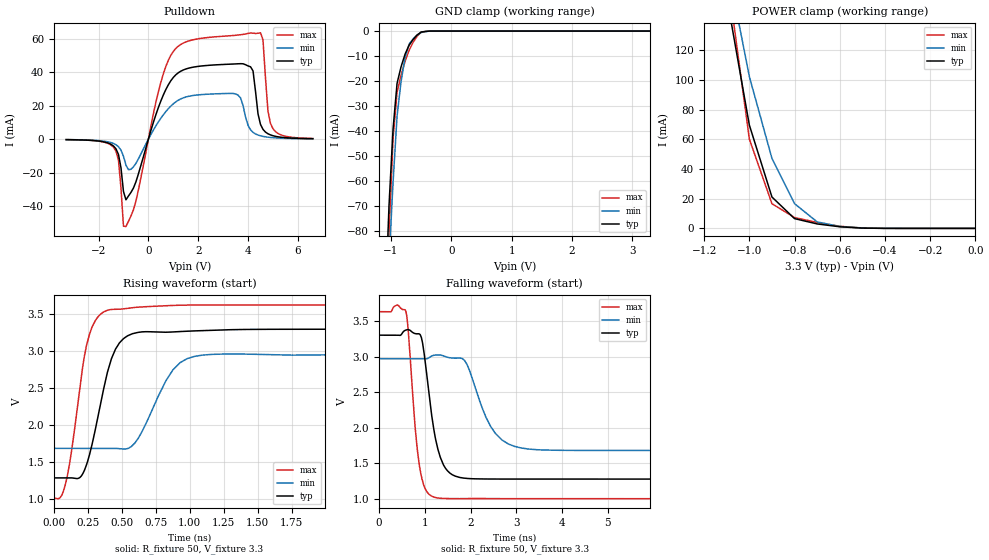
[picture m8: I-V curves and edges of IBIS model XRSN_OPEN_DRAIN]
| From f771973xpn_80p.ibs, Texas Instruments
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|   Model Cell XRSN_OPEN_DRAIN
|XRSN_OPEN_DRAIN
[Model]   XRSN_OPEN_DRAIN
Model_type   I/O_open_drain
Polarity   Non-Inverting
Enable   Active-High
Vinl =  0.8
Vinh =  2
Cref =  15.0000pF
Rref =  100.0000M
Vref =  0V
Vmeas =  1.65
C_comp   4.25494p   0.807076p   4.29559p
[Model Spec]
Vinl   0.8   0.8   0.8
Vinh   2   2   2
[Temperature Range]   25   155   -40
[Voltage Range]   3.3   2.97   3.63
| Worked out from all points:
|   slope of the pulldown table from 0 to 0.495 V, typ, clamps not added: 22 ohm
|   GND clamp passes 1 mA (typ) near -0.53 V on its own axis
|   POWER clamp passes 1 mA (typ) near -0.59 V on its own axis
|   rising waveform, R_fixture 50, V_fixture 3.3: 20-80 % time 149ps typ, 207ps min, 123ps max; typ from 1.28 V to 3.3 V
|   falling waveform, R_fixture 50, V_fixture 3.3: 20-80 % time 278ps typ, 497ps min, 202ps max; typ from 3.3 V to 1.28 V
| Nom Voltages:
|   BIASFET=3.3, VDD=1.2, VDDS=3.3, VSS=0
| Min Voltages:
|   BIASFET=2.97, VDD=1.08, VDDS=2.97, VSS=0
| Max Voltages:
|   BIASFET=3.63, VDD=1.32, VDDS=3.63, VSS=0
[POWER_clamp]
|   voltage   I(typ)   I(min)   I(max)
-3.3V     2.375A     2.63A      3.153A
-1.1V     156mA      180.1mA    173.4mA
-1.067V   127.2mA    154.1mA    135.6mA
-1.033V   98.41mA    128.2mA    97.92mA
-1V       69.61mA    102.3mA    60.2mA
-900mV    21.13mA    47.13mA    16.61mA
-800mV    6.576mA    16.63mA    7.309mA
-700mV    2.999mA    4.377mA    3.99mA
-600mV    1.087mA    1.246mA    1.425mA
-500mV    187uA      310uA      203.4uA
0V        311.4pA    5.945nA    272.3pA
[Pulldown]
|   voltage   I(typ)   I(min)   I(max)
-3.3V     -269.8uA   -248.1uA   -260.2uA
-1.4V     -4.056mA   -2.548mA   -4.78mA
-1.2V     -9.104mA   -4.482mA   -12.53mA
-900mV    -36.12mA   -15.43mA   -52.08mA
1V        36.78mA    21.07mA    52.28mA
3.5V      44.86mA    26.98mA    61.93mA
4.1V      43.14mA    5.597mA    63.29mA
4.5V      8.805mA    2.015mA    63.4mA
4.6V      5.861mA    1.67mA     59.29mA
4.8V      3.241mA    1.198mA    16.69mA
5V        2.072mA    897.2uA    6.272mA
6.6V      302.2uA    231.8uA    414.2uA
[GND_clamp]
|   voltage   I(typ)   I(min)   I(max)
-3.3V     -1.947A    -1.623A    -3.254A
-1.1V     -112mA     -127mA     -135.8mA
-1.033V   -69.61mA   -91.63mA   -80.19mA
-966.7mV  -39.23mA   -60.62mA   -43.11mA
-900mV    -20.86mA   -34.02mA   -24.52mA
-833.3mV  -14.26mA   -20.12mA   -17.61mA
-766.7mV  -9.194mA   -10.52mA   -12.01mA
-700mV    -5.668mA   -5.208mA   -7.706mA
-566.7mV  -1.566mA   -1.573mA   -2.055mA
-500mV    -402.3uA   -585.8uA   -459.7uA
-300mV    -821.9nA   -7.169uA   -404.6nA
3.3V      311.4pA    8.957uA    217.5pA
[Ramp]
| variable   typ   min   max
dV/dt_f  1.2593654/0.28302832n 0.80461726/0.50819432n  1.6314999/0.2056677n
dV/dt_r  1.2022968/0.27309132n 0.74728283/0.51227243n  1.5167269/0.19733027n
R_load = 50
[Rising Waveform]
R_fixture = 50
V_fixture = 3.3
V_fixture_min = 2.97
V_fixture_max = 3.63
|   time   V(typ)   V(min)   V(max)
0s        1.281V     1.682V     1.005V
90ps      1.281V     1.682V     1.228V
202.1ps   1.305V     1.682V     2.654V
282.4ps   1.743V     1.682V     3.333V
394.3ps   2.714V     1.683V     3.557V
454ps     3.029V     1.681V     3.571V
639.4ps   3.261V     1.876V     3.602V
876.9ps   3.263V     2.749V     3.623V
1.216ns   3.289V     2.962V     3.63V
20.01ns   3.3V       2.97V      3.63V
[Falling Waveform]
R_fixture = 50
V_fixture = 3.3
V_fixture_min = 2.97
V_fixture_max = 3.63
|   time   V(typ)   V(min)   V(max)
0s        3.3V       2.97V      3.63V
588.6ps   3.372V     2.97V      3.633V
886.7ps   3.314V     2.97V      1.456V
1.018ns   2.885V     2.967V     1.134V
1.272ns   1.736V     3.023V     1.016V
1.657ns   1.324V     2.977V     1.006V
1.922ns   1.29V      2.891V     1.007V
2.548ns   1.281V     1.917V     1.006V
3.269ns   1.281V     1.702V     1.005V
20.01ns   1.281V     1.682V     1.005V
